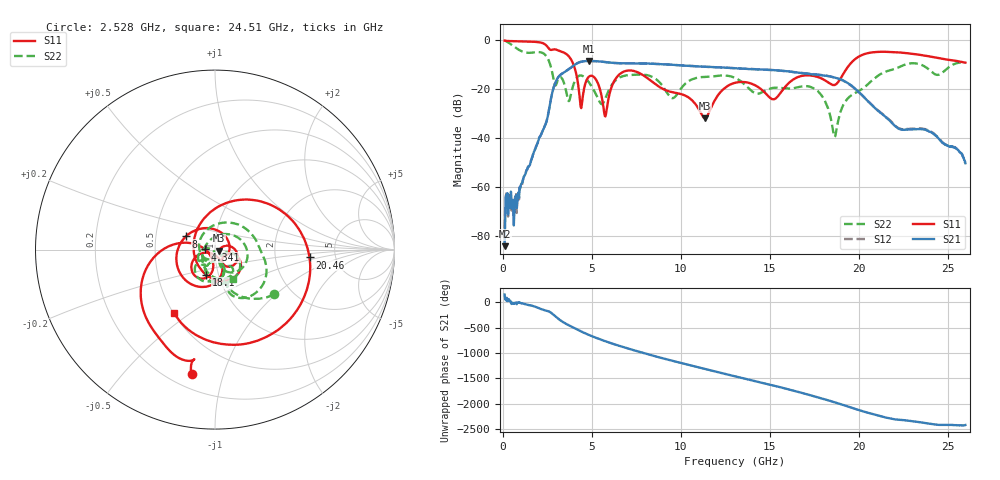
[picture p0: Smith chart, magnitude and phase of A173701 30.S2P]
!  2-Port S-parameters saved by WinCal
! VAR MeasName=S-Parameters (CALIBRATED_DATA) read from VNA (N5245A)
! VAR MeasDate=2017-6-7 10:30:22
! VAR NAME=A173701 30
! VAR FILENAME=A173701 30.S2P
! VAR DATE=2017-6-7 10:30:22
! VAR PHYS_PORTS=1,2
# Hz S DB R 50
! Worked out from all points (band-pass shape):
!   801 points, 100 MHz to 26 GHz, reference 50 ohm
!   highest |S21| = -8.65 dB at 4.859 GHz (marker M1); lowest = -84.3 dB at 100 MHz (marker M2)
!   |S21| within 3 dB of the highest: 3.771 GHz to 13.16 GHz (9.39 GHz wide, 111 % of centre)
!   lowest |S11| = -32.0 dB at 11.37 GHz (marker M3), VSWR 1.05, Z = 52.5 - j0.634 ohm
!   |S11| at or under -10 dB: 3.964 GHz to 19.51 GHz (15.55 GHz wide, 132 % of centre)
!   |S22| runs from -39.6 to -0.3 dB; largest |S21 - S12| = 0.0039
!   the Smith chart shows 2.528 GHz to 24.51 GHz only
!   S11 on the Smith chart (normalised r, x): 2.528 GHz: 0.29, -0.79; 4.341 GHz: 0.89, +0.00; 8 GHz: 0.71, +0.11; 18.1 GHz: 0.87, -0.25; 20.46 GHz: 3.19, -0.39; 24.51 GHz: 0.50, -0.43
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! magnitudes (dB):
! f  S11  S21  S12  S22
! 100 MHz  -0.3  -84.3  -77.0  -0.3
! 2.528 GHz  -3.0  -31.2  -31.1  -7.7
! 2.981 GHz  -4.0  -17.0  -17.0  -18.6
! 3.694 GHz  -6.6  -12.1  -12.0  -25.0
! 4.341 GHz  -25.1  -9.1  -9.1  -14.6
! 4.438 GHz  -26.6  -8.9  -8.9  -14.6
! 4.859 GHz  -15.0  -8.7  -8.6  -17.6
! 5.766 GHz  -31.3  -9.1  -9.1  -23.9
! 6.575 GHz  -14.0  -9.6  -9.6  -15.3
! 8 GHz  -15.0  -9.6  -9.7  -14.3
! 8.744 GHz  -19.0  -9.9  -9.9  -16.9
! 9.553 GHz  -21.4  -10.2  -10.2  -23.8
! 11.37 GHz  -32.0  -11.0  -11.0  -15.2
! 13.05 GHz  -17.6  -11.6  -11.6  -15.6
! 15.22 GHz  -24.3  -12.4  -12.4  -19.6
! 17.39 GHz  -14.6  -14.1  -14.0  -19.5
! 18.1 GHz  -16.5  -14.7  -14.6  -24.9
! 18.65 GHz  -18.5  -15.4  -15.4  -39.6
! 20.46 GHz  -5.5  -24.7  -24.6  -18.5
! 21.69 GHz  -4.9  -32.7  -32.5  -12.6
! 24.51 GHz  -7.5  -40.5  -40.2  -14.2
! 26 GHz  -9.3  -50.4  -50.1  -9.3
